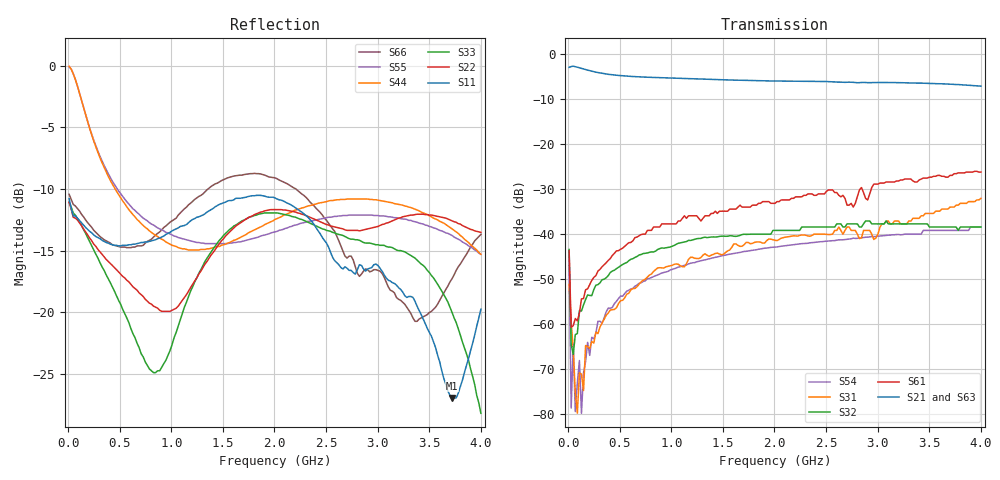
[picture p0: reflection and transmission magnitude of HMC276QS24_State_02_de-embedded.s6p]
! Hittite Microwave Corporation
! 20 Alpha Road
! Chelmsford, MA 01824
! Tel: 978-250-3343
! Fax: 978-250-3373
! Device: HMC276QS24, 0.7-3.0 GHz, GaAS MMIC 4x2 Switch Matrix in 24-lead QSOP package
! Misc: Data was de-embedded to package pins.
!  Port 1 = OP1
!  Port 2 = VL
!  Port 3 = VH
!  Port 4 = HH
!  Port 5 = HL
!  Port 6 = OP2
!  Vdd = +5 V
!  Vctl = 0 V[Logic 0] / +5 V[Logic 1]
!  State 02,  VL to OP1,  VH to OP2
!  Control Lines (Logic)
!  HV 1 = 0, Tone 1 = 0
!  HV 2 = 0, Tone 2 = 1
!  Data reformated to new Touchstone file format - Wed Jan 10 14:22:19 2007
# MHz S DB R 50
! 6 Port Network Data
! freq  dbS11  angS11  dbS12  angS12  dbS13  angS13  dbS14  angS14
!  dbS15  angS15  dbS16  angS16
!  dbS21  angS21  dbS22  angS22
!  dbS23  angS23  dbS24  angS24  dbS25  angS25  dbS26  angS26
!  dbS31  angS31  dbS32  angS32  dbS33  angS33  dbS34  angS34
!  dbS35  angS35  dbS36  angS36
!  dbS41  angS41  dbS42  angS42
!  dbS43  angS43  dbS44  angS44  dbS45  angS45  dbS46  angS46
!  dbS51  angS51  dbS52  angS52  dbS53  angS53  dbS54  angS54
!  dbS55  angS55  dbS56  angS56
!  dbS61  angS61  dbS62  angS62
!  dbS63  angS63  dbS64  angS64  dbS65  angS65  dbS66  angS66
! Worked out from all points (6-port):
!   201 points, 10 MHz to 4 GHz, reference 50 ohm
!   strongest paths, dB at 10 MHz, 1.008 GHz, 2.005 GHz, 3.002 GHz, 4 GHz:
!     S21: -2.9, -5.3, -5.9, -6.3, -7.1
!     S63: -2.8, -5.4, -6.0, -6.1, -6.9
!     S61: -43.7, -37.7, -33.2, -28.9, -26.2
!     S32: -43.4, -42.7, -39.2, -37.7, -38.4
!     S31: -51.2, -46.9, -41.4, -40.0, -32.0
!     S54: -46.9, -47.8, -42.9, -40.5, -38.4
!   lowest |S11| = -26.9 dB at 3.721 GHz (marker M1), VSWR 1.09, Z = 48.8 + j4.29 ohm
!   |S11| at or under -10 dB: start of sweep to end of sweep
